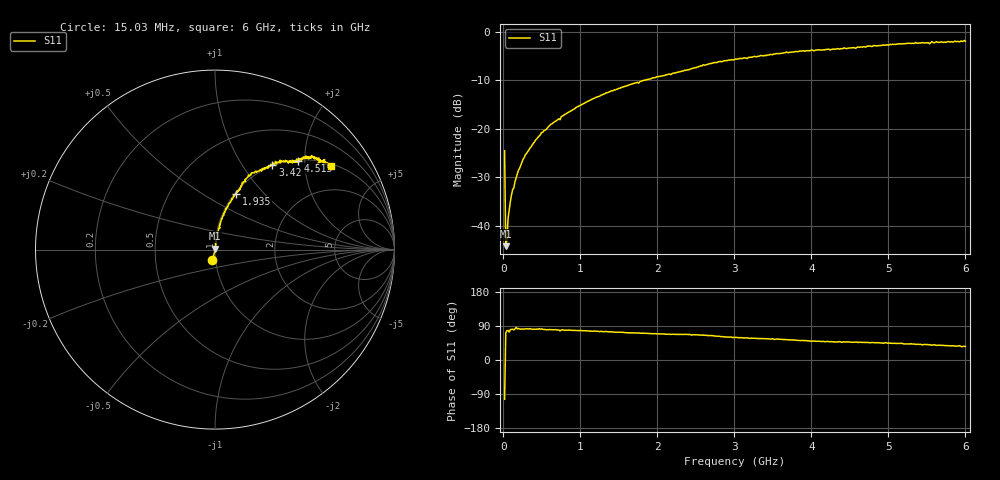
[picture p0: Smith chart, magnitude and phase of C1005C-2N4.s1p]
!	Network	Analyzer	HP8753E.07.74:	Oct	30	2002	Serial	No.	JP38451487
!	Hewlett-Packard
!	7	Sep	2009	8:19:55
!	Frequency	S11
#	HZ	S	RI	R	50
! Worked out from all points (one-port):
!   400 points, 15.03 MHz to 6 GHz, reference 50 ohm
!   lowest |S11| = -44.3 dB at 30.03 MHz (marker M1), VSWR 1.01, Z = 50.2 + j0.581 ohm
!   |S11| at or under -10 dB: start of sweep to 1.84 GHz
!   S11 on the Smith chart (normalised r, x): 15.03 MHz: 0.97, -0.11; 1.935 GHz: 1.01, +0.71; 3.42 GHz: 0.98, +1.38; 4.515 GHz: 1.01, +1.86; 6 GHz: 1.07, +2.73
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1.502992e7  -0.014 -0.0574
3.002985e7  0.00199 0.00579
4.502978e7  0.00153 0.00693
6.00297e7  0.00247 0.0116
1.050295e8  0.00331 0.0205
1.95029e8  0.00448 0.0369
2.550287e8  0.00712 0.0477
4.950275e8  0.0125 0.0903
7.350263e8  0.0281 0.12
7.650262e8  0.0234 0.133
1.155024e9  0.0496 0.196
1.515022e9  0.0751 0.25
1.93502e9  0.117 0.312
2.265019e9  0.144 0.354
3.015015e9  0.263 0.452
3.420013e9  0.32 0.474
3.765011e9  0.371 0.492
4.515007e9  0.464 0.496
5.265004e9  0.562 0.512
5.445003e9  0.592 0.495
5.535002e9  0.573 0.48
5.565002e9  0.611 0.502
5.595002e9  0.585 0.495
5.625002e9  0.616 0.49
5.865001e9  0.64 0.476
5.925e9  0.62 0.481
5.955e9  0.653 0.45
6e9  0.647 0.466
